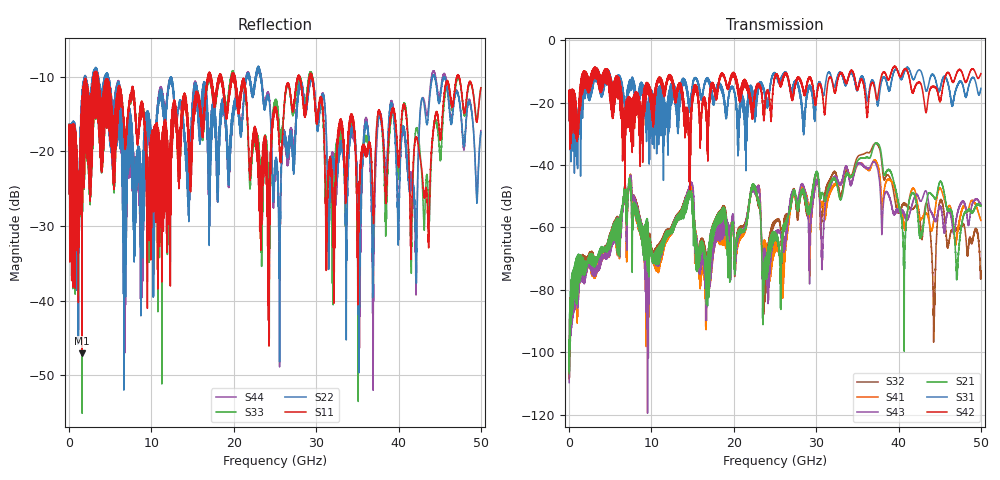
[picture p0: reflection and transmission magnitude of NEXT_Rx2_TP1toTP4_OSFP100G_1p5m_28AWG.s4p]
! Touchstone data
! Created: 27-Feb-2019 by IdEM 12 (12.1.0)
! COMMENTS
!  Created Wed Feb 27 09:43:39 2019
!  64 Port Network Data from SP1.SP block
!  freq  magS1_1  angS1_1  magS1_2  angS1_2  magS1_3  angS1_3  magS1_4  angS1_4
!  magS1_5  angS1_5  magS1_6  angS1_6  magS1_7  angS1_7  magS1_8  angS1_8
!  magS1_9  angS1_9  magS1_10  angS1_10  magS1_11  angS1_11  magS1_12  angS1_12
!  magS1_13  angS1_13  magS1_14  angS1_14  magS1_15  angS1_15  magS1_16  angS1_16
!  magS1_17  angS1_17  magS1_18  angS1_18  magS1_19  angS1_19  magS1_20  angS1_20
!  magS1_21  angS1_21  magS1_22  angS1_22  magS1_23  angS1_23  magS1_24  angS1_24
!  magS1_25  angS1_25  magS1_26  angS1_26  magS1_27  angS1_27  magS1_28  angS1_28
!  magS1_29  angS1_29  magS1_30  angS1_30  magS1_31  angS1_31  magS1_32  angS1_32
!  magS1_33  angS1_33  magS1_34  angS1_34  magS1_35  angS1_35  magS1_36  angS1_36
!  magS1_37  angS1_37  magS1_38  angS1_38  magS1_39  angS1_39  magS1_40  angS1_40
!  magS1_41  angS1_41  magS1_42  angS1_42  magS1_43  angS1_43  magS1_44  angS1_44
!  magS1_45  angS1_45  magS1_46  angS1_46  magS1_47  angS1_47  magS1_48  angS1_48
!  magS1_49  angS1_49  magS1_50  angS1_50  magS1_51  angS1_51  magS1_52  angS1_52
!  magS1_53  angS1_53  magS1_54  angS1_54  magS1_55  angS1_55  magS1_56  angS1_56
!  magS1_57  angS1_57  magS1_58  angS1_58  magS1_59  angS1_59  magS1_60  angS1_60
!  magS1_61  angS1_61  magS1_62  angS1_62  magS1_63  angS1_63  magS1_64  angS1_64
!  magS2_1  angS2_1  magS2_2  angS2_2  magS2_3  angS2_3  magS2_4  angS2_4
!  magS2_5  angS2_5  magS2_6  angS2_6  magS2_7  angS2_7  magS2_8  angS2_8
!  magS2_9  angS2_9  magS2_10  angS2_10  magS2_11  angS2_11  magS2_12  angS2_12
!  magS2_13  angS2_13  magS2_14  angS2_14  magS2_15  angS2_15  magS2_16  angS2_16
!  magS2_17  angS2_17  magS2_18  angS2_18  magS2_19  angS2_19  magS2_20  angS2_20
!  magS2_21  angS2_21  magS2_22  angS2_22  magS2_23  angS2_23  magS2_24  angS2_24
!  magS2_25  angS2_25  magS2_26  angS2_26  magS2_27  angS2_27  magS2_28  angS2_28
!  magS2_29  angS2_29  magS2_30  angS2_30  magS2_31  angS2_31  magS2_32  angS2_32
!  magS2_33  angS2_33  magS2_34  angS2_34  magS2_35  angS2_35  magS2_36  angS2_36
!  magS2_37  angS2_37  magS2_38  angS2_38  magS2_39  angS2_39  magS2_40  angS2_40
!  magS2_41  angS2_41  magS2_42  angS2_42  magS2_43  angS2_43  magS2_44  angS2_44
!  magS2_45  angS2_45  magS2_46  angS2_46  magS2_47  angS2_47  magS2_48  angS2_48
!  magS2_49  angS2_49  magS2_50  angS2_50  magS2_51  angS2_51  magS2_52  angS2_52
!  magS2_53  angS2_53  magS2_54  angS2_54  magS2_55  angS2_55  magS2_56  angS2_56
!  magS2_57  angS2_57  magS2_58  angS2_58  magS2_59  angS2_59  magS2_60  angS2_60
!  magS2_61  angS2_61  magS2_62  angS2_62  magS2_63  angS2_63  magS2_64  angS2_64
!  magS3_1  angS3_1  magS3_2  angS3_2  magS3_3  angS3_3  magS3_4  angS3_4
!  magS3_5  angS3_5  magS3_6  angS3_6  magS3_7  angS3_7  magS3_8  angS3_8
!  magS3_9  angS3_9  magS3_10  angS3_10  magS3_11  angS3_11  magS3_12  angS3_12
!  magS3_13  angS3_13  magS3_14  angS3_14  magS3_15  angS3_15  magS3_16  angS3_16
!  magS3_17  angS3_17  magS3_18  angS3_18  magS3_19  angS3_19  magS3_20  angS3_20
!  magS3_21  angS3_21  magS3_22  angS3_22  magS3_23  angS3_23  magS3_24  angS3_24
!  magS3_25  angS3_25  magS3_26  angS3_26  magS3_27  angS3_27  magS3_28  angS3_28
!  magS3_29  angS3_29  magS3_30  angS3_30  magS3_31  angS3_31  magS3_32  angS3_32
!  magS3_33  angS3_33  magS3_34  angS3_34  magS3_35  angS3_35  magS3_36  angS3_36
!  magS3_37  angS3_37  magS3_38  angS3_38  magS3_39  angS3_39  magS3_40  angS3_40
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# Hz S MA R 50
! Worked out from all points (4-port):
!   5000 points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, 10 MHz to 50 GHz, reference 50 ohm
!   strongest paths, dB at 10 MHz, 12.51 GHz, 25.01 GHz, 37.51 GHz, 50 GHz:
!     S42: -19.6, -12.4, -11.6, -17.8, -10.7
!     S31: -19.6, -16.2, -10.8, -21.0, -15.4
!     S21: -106.9, -61.0, -62.9, -33.2, -53.1
!     S43: -109.7, -60.6, -63.2, -41.9, -52.6
!     S41: -108.6, -61.4, -66.2, -40.2, -57.8
!     S32: -108.2, -60.3, -58.7, -33.7, -76.5
!   lowest |S11| = -47.1 dB at 1.59 GHz (marker M1), VSWR 1.01, Z = 49.7 + j0.298 ohm
!   |S11| at or under -10 dB: 3.482 GHz to 16.85 GHz (13.37 GHz wide, 132 % of centre); 20.15 GHz to 27.79 GHz (7.635 GHz wide, 31.9 % of centre); 29.53 GHz to 47.08 GHz (17.55 GHz wide, 45.8 % of centre)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
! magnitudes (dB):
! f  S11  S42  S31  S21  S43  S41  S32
! 10 MHz  -19.2  -19.6  -19.6  -106.9  -109.7  -108.6  -108.2
! 1.59 GHz  -47.1  -17.4  -24.2  -69.7  -70.8  -71.2  -68.9
! 22.4 GHz  -17.3  -21.8  -20.3  -46.1  -46.9  -46.4  -46.6
! 23.68 GHz  -20.5  -25.8  -16.8  -72.7  -66.7  -64.1  -86.8
! 37.22 GHz  -19.8  -17.2  -16.6  -33.0  -39.5  -38.5  -33.0
! 40.65 GHz  -13.7  -9.4  -10.5  -79.3  -56.0  -58.8  -52.1
! 50 GHz  -11.5  -10.7  -15.4  -53.1  -52.6  -57.8  -76.5
